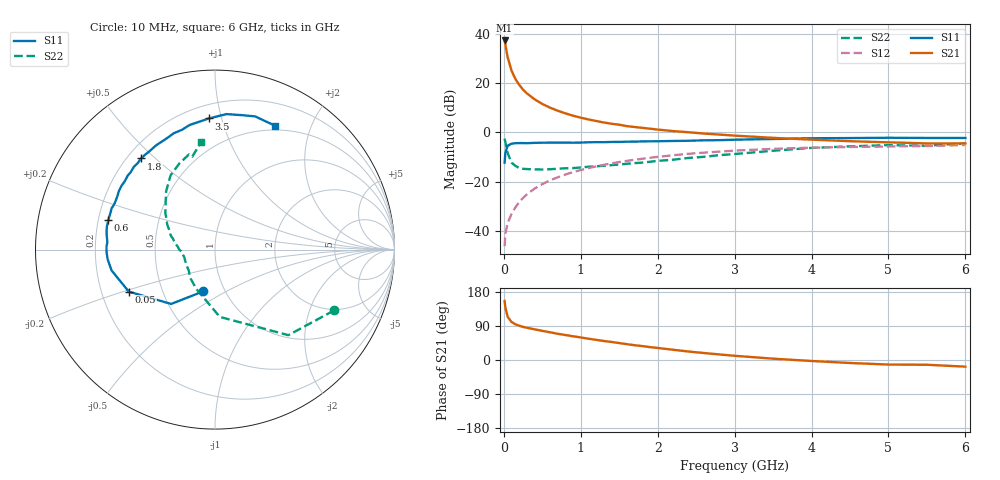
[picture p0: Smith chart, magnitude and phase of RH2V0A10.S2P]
! SIEMENS Small Signal Semiconductors
! BFR106
! Si NPN RF Bipolar Junction Transistor in SOT23
! VCE = 2 V  IC = 100 mA
! Common Emitter S-Parameters:  August  1996
# GHz  S  MA  R  50
!  f  S11  S21  S12  S22
! GHz  MAG  ANG  MAG  ANG  MAG  ANG  MAG  ANG
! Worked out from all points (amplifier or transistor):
!   36 points, 10 MHz to 6 GHz, reference 50 ohm
!   highest |S21| = 37.3 dB at 10 MHz (marker M1)
!   |S21| within 3 dB of that: start of sweep to 27.12 MHz
!   unconditionally stable (mu >= 1): 112 MHz to end of sweep
!   at 250 MHz: K = 1.14, MAG = 19.7 dB, |S12| = -26.6 dB
!   at 1.4 GHz: K = 1.11, MAG = 6.0 dB, |S12| = -12.6 dB
!   at 6 GHz: K = 1.02, MAG = -0.6 dB, |S12| = -5.2 dB
!   S11 on the Smith chart (normalised r, x): 10 MHz: 0.79, -0.39; 50 MHz: 0.32, -0.21; 600 MHz: 0.24, +0.13; 1.8 GHz: 0.25, +0.45; 3.5 GHz: 0.29, +0.91; 6 GHz: 0.45, +1.50
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0.01  0.2421 -105.8  72.98 155.7  0.0049 71.3  0.7447 -27.1
0.02  0.3891 -128.9  59.4 138.3  0.0088 64.4  0.6279 -49.4
0.05  0.5341 -154.0  32.99 113.8  0.0145 58.5  0.376 -85.9
0.1  0.588 -168.6  17.83 100.4  0.0221 64.6  0.2429 -115.3
0.15  0.6008 -175.0  12.09 94.2  0.03 68.8  0.2089 -131.7
0.2  0.6043 -178.6  9.18 90.4  0.0386 71.3  0.1881 -140.8
0.25  0.6048 178.4  7.339 87.3  0.0467 72.4  0.1817 -149.0
0.3  0.6012 176.0  6.152 85.1  0.0554 73.3  0.1796 -153.3
0.4  0.6111 171.5  4.671 80.9  0.0722 73.5  0.177 -160.9
0.5  0.6157 168.2  3.761 76.9  0.0889 73.0  0.1759 -165.6
0.6  0.6169 164.7  3.164 73.1  0.1058 71.8  0.178 -168.5
0.7  0.6171 161.3  2.743 69.2  0.1224 70.5  0.1828 -171.3
0.8  0.6202 158.3  2.42 66.0  0.1391 69.1  0.1862 -174.5
1.1  0.6273 148.5  1.825 56.2  0.1881 64.3  0.2003 179.6
1.4  0.6374 139.7  1.492 47.6  0.2341 59.0  0.2157 173.4
1.8  0.6543 129.1  1.231 36.7  0.2905 51.9  0.2427 165.2
2.2  0.6675 119.3  1.059 27.0  0.3428 44.9  0.2781 156.7
2.8  0.6923 105.4  0.9 14.7  0.4064 34.4  0.3437 143.6
3.5  0.7317 92.6  0.772 3.5  0.4626 23.2  0.4231 130.1
4.5  0.7639 78.7  0.66 -7.9  0.5031 8.9  0.5188 112.6
5.5  0.7678 67.9  0.595 -12.6  0.5259 0.4  0.5324 103.8
6  0.7676 64.1  0.595 -17.5  0.5522 -6.2  0.6048 97.3
